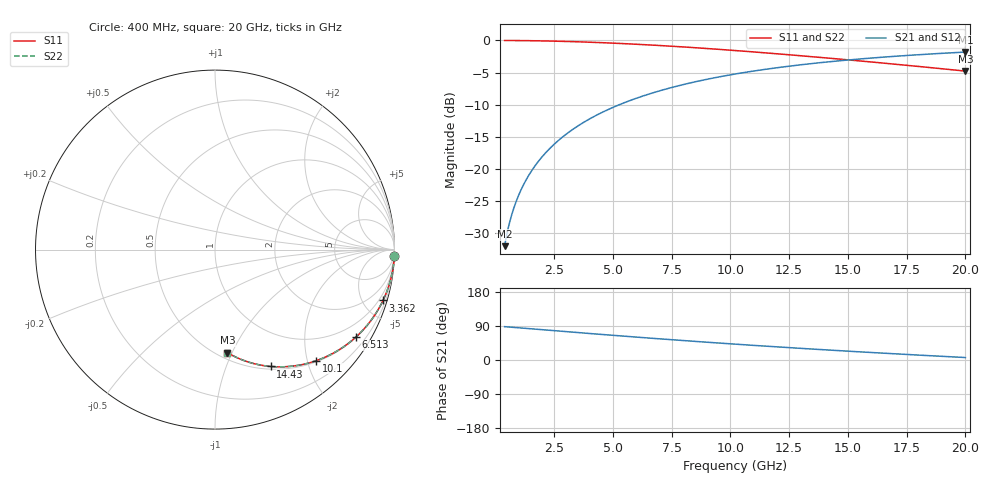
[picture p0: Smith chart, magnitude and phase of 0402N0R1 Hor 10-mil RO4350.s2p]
# GHz S MA R 50
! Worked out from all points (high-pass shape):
!   1960 points, 400 MHz to 20 GHz, reference 50 ohm
!   highest |S21| = -1.81 dB at 20 GHz (marker M1); lowest = -32.0 dB at 400 MHz (marker M2)
!   |S21| within 3 dB of the highest: 10.9 GHz to end of sweep
!   lowest |S11| = -4.8 dB at 20 GHz (marker M3), VSWR 3.73, Z = 27.9 - j47.9 ohm
!   |S11| at or under -10 dB: nowhere
!   |S22| runs from -4.8 to 0.0 dB; largest |S21 - S12| = 0
!   S11 on the Smith chart (normalised r, x): 400 MHz: 1, -57; 3.362 GHz: 0.51, -6.71; 6.513 GHz: 0.51, -3.43; 10.1 GHz: 0.52, -2.16; 14.43 GHz: 0.53, -1.45; 20 GHz: 0.56, -0.96
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0.4  0.9997 -2.0  0.02513 88.0  0.02513 88.0  0.9997 -2.0
0.4600306  0.9996 -2.3  0.02889 87.7  0.02889 87.7  0.9996 -2.3
0.6501276  0.9991 -3.3  0.04082 86.7  0.04082 86.7  0.9991 -3.3
0.8502297  0.9985 -4.3  0.05335 85.7  0.05335 85.7  0.9985 -4.3
1.110362  0.9975 -5.6  0.06961 84.4  0.06961 84.4  0.9975 -5.6
1.430526  0.9959 -7.2  0.08955 82.8  0.08955 82.8  0.9959 -7.2
1.81072  0.9935 -9.1  0.1131 80.9  0.1131 80.9  0.9935 -9.1
2.260949  0.9899 -11.4  0.1408 78.6  0.1408 78.6  0.9899 -11.4
2.77121  0.985 -13.9  0.1718 76.1  0.1718 76.1  0.985 -13.9
3.361511  0.9781 -16.9  0.2071 73.1  0.2071 73.1  0.9781 -16.9
3.671669  0.974 -18.4  0.2253 71.6  0.2253 71.6  0.974 -18.4
4.962328  0.9538 -24.6  0.299 65.3  0.299 65.3  0.9538 -24.6
6.513119  0.9237 -31.9  0.3815 58.0  0.3815 58.0  0.9237 -31.9
6.943338  0.9144 -33.9  0.4031 56.1  0.4031 56.1  0.9144 -33.9
8.504135  0.878 -40.8  0.4767 49.1  0.4767 49.1  0.878 -40.8
10.10495  0.8374 -47.7  0.5442 42.2  0.5442 42.2  0.8374 -47.7
10.205  0.8348 -48.1  0.5482 41.8  0.5482 41.8  0.8348 -48.1
11.78581  0.7929 -54.5  0.6066 35.4  0.6066 35.4  0.7929 -54.5
13.46667  0.7477 -60.9  0.661 28.9  0.661 28.9  0.7477 -60.9
14.42716  0.7219 -64.4  0.6888 25.4  0.6888 25.4  0.7219 -64.4
16.73834  0.6606 -72.6  0.747 17.2  0.747 17.2  0.6606 -72.6
20  0.5776 -83.2  0.812 6.5  0.812 6.5  0.5776 -83.2
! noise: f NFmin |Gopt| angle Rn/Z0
0.4  0.006145  0.9752  1.994  0.0563
2.571  0.007848  0.8556  10.64  0.01151
4.752  0.01001  0.7678  16.13  0.008605
6.933  0.01222  0.7063  20.04  0.007936
9.104  0.01439  0.6622  23.25  0.007837
11.29  0.01653  0.6289  26.15  0.007948
13.47  0.01863  0.6029  28.89  0.008153
15.64  0.0207  0.5821  31.53  0.008403
17.82  0.02276  0.565  34.13  0.008678
20  0.02481  0.5508  36.69  0.008966
